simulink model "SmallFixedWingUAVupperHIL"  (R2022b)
settings: Solver=FixedStepDiscrete  StartTime=0.0  StopTime=stoptime  RelTol=1e-3
model workspace: external: MAT-File (data not in the file)
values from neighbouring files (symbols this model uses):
  env = struct    [InitDatactrl.m]
  stoptime = knots(m-pp+1)    [bspline.m]    (also in generate_poly.m = 20)
  uav = struct    [InitDatactrl.m]    (also in InitDatactrldf.m)
  x = x + points(1, i) * k(i) * ft    [bezir_n.m]
undefined symbols (not defined in the file or in its folder): current_a, current_filtered_a, DiscIntNeverNeededParam, remaining, RGBLED_COLOR_ENUM, RGBLED_MODE_ENUM, voltage_filtered_v, voltage_v
libraries: simulink x9, pixhawk_slib_sensors_actuators x4, pixhawk_slib_uORB_RW x3

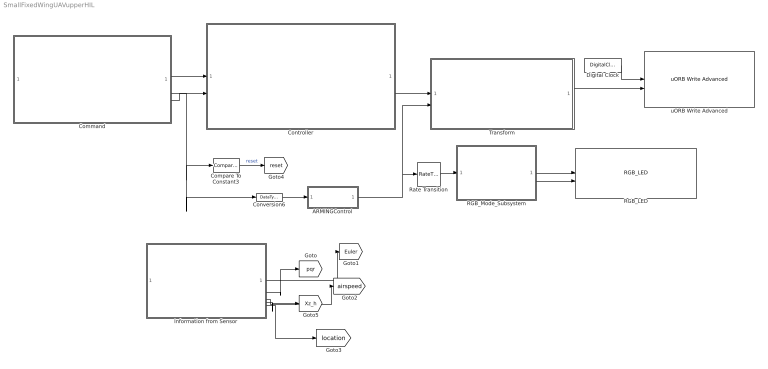
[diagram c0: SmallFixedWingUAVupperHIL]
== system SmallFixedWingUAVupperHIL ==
  ARMINGControl : Subsystem
  Command : Subsystem
  Compare To Constant3 : simulink/Logic and Bit Operations/Compare To Constant  relop=<=  const=1100  OutDataTypeStr=boolean
  Controller : Subsystem
  Conversion6 : DataTypeConversion  OutDataTypeStr=double
  Digital Clock : DigitalClock  SampleTime=-1
  Information from Sensor : Subsystem
  RGB_LED : pixhawk_slib_sensors_actuators/RGB_LED
  RGB_Mode_Subsystem : Subsystem
  Rate Transition : RateTransition  OutPortSampleTime=1
  Transform : Subsystem
  uORB Write Advanced : pixhawk_slib_uORB_RW/uORB Write Advanced  Ts=0  uORB_AdvtQueue=on  uORB_FieldEnabledArr="0  0  0  1  0  0  0  0  0  0  0"  uORB_Topic_str=0  uORB_Struct_DT="[1  1  1  1  1]"  BlockInputCount=5  uORB_StructParams="[\"voltage_v\",\"voltage_filtered_v\",\"current_a\",\"current_filtered_a\",\"remaining\"]"  uORB_PortSizes="[1  1  1  1]"  MsgSizeOf=0  MW_update=true
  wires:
  Digital Clock/1 -> uORB Write Advanced/1
  RGB_Mode_Subsystem/1(RGB_MODE) -> RGB_LED/1
  Rate Transition/1 -> RGB_Mode_Subsystem/1(ARM_STATE)
  ARMINGControl/1(Out1) -> Transform/2(In2), Rate Transition/1
  RGB_Mode_Subsystem/2(RGB_COLOR) -> RGB_LED/2
  Conversion6/1 -> ARMINGControl/1(In1)
  Compare To Constant3/1 -> [reset]  "reset"
  Transform/1(Out1) -> uORB Write Advanced/2
  Controller/1(Out1) -> Transform/1(In1)
  Command/2(Arm) -> Conversion6/1, Compare To Constant3/1
  Command/1(Command) -> Controller/1(Cmd)
  Information from Sensor/2(pqr) -> [pqr]
  Information from Sensor/4(Xz_h) -> [Xz_h]
  Information from Sensor/3(<true_airspeed_m_s>) -> [airspeed]
  Information from Sensor/1(Euler) -> [Euler]
  Information from Sensor/5(location) -> [location]
  Command/3(Command1) -> Controller/2(Cmd1)

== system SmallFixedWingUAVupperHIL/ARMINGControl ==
  In1 : Inport
  Compare To Constant3 : simulink/Logic and Bit Operations/Compare To Constant  relop=>=  const=uint16(1500)  OutDataTypeStr=boolean
  Out1 : Outport  VectorParamsAs1DForOutWhenUnconnected=off
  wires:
  Compare To Constant3/1 -> Out1/1
  In1/1 -> Compare To Constant3/1

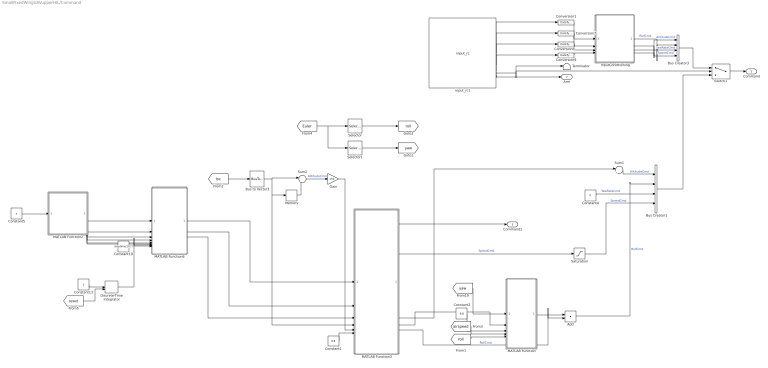
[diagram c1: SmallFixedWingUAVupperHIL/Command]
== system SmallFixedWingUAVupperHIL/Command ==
  Add : Sum
  Bus Creator1 : BusCreator  Inputs=4
  Bus Creator3 : BusCreator  Inputs=4
  Bus to Vector3 : BusToVector
  Constant1 : Constant  Value=9.8
  Constant13 : Constant  SampleTime=-1
  Constant19 : Constant  Value=stoptime/1000
  Constant2 : Constant  Value=9.8  SampleTime=-1
  Constant4 : Constant  Value=0  SampleTime=-1
  Constant5 : Constant  Value=x
  Conversion{1,7..9} (4 alike) : DataTypeConversion  OutDataTypeStr=double
  Discrete-Time Integrator : DiscreteIntegrator  ExternalReset=either  SampleTime=-1  ICPrevOutput=DiscIntNeverNeededParam  ICPrevScaledInput=DiscIntNeverNeededParam
  Gain : Gain  Gain=150
  InputConditioning : Subsystem
  MATLAB Function : MATLAB Function  TreatAsAtomicUnit=on
  MATLAB Function2 : MATLAB Function  TreatAsAtomicUnit=on
  MATLAB Function3 : MATLAB Function  TreatAsAtomicUnit=on
  MATLAB Function6 : MATLAB Function  TreatAsAtomicUnit=on
  Memory : Memory  InheritSampleTime=on
  Saturation : Saturate  UpperLimit=15  LowerLimit=10
  Selector : Selector  InputPortWidth=3  IndexOptions=Index vector (dialog)  Indices=[1]  OutputSizes=1
  Selector1 : Selector  InputPortWidth=3  IndexOptions=Index vector (dialog)  Indices=[3]  OutputSizes=1
  Sum1 : Sum  Inputs=|++
  Sum2 : Sum  Inputs=|+-
  Switch1 : Switch  Criteria=u2 > Threshold  Threshold=1500
  Terminator : Terminator
  input_rc1 : pixhawk_slib_sensors_actuators/input_rc  Description=|  sampletime=1/250  channel1=on  channel2=on  channel3=on  channel4=on  channel5=on  channel6=on  channel7=off  channel8=off  channel9=off  channel10=off  channel11=off  channel12=off  channel13=off  channel14=off  channel15=off  channel16=off  channel17=off  channel18=off  ch_count=off  rssi=off  rc_failsafe=off  rc_lost=off  rc_inputsource=off
      | RC Input Block
      | 
      | This block provides user input control to the model.
      | It uses the input_rc uORB topic.
      | 
      | The user has the ability to choose which channels are available as outputs from this block and also some optional outputs. These include 
      | Channels 1 through 18
      | double data type indicating the PWM value from the controller 
      | measured pulse widths for each of the supported channels 
      | Channel Count 
      | u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
  Command : Outport  VectorParamsAs1DForOutWhenUnconnected=off
  Arm : Outport  Port=2  VectorParamsAs1DForOutWhenUnconnected=off
  Command1 : Outport  Port=3  VectorParamsAs1DForOutWhenUnconnected=off
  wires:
  InputConditioning/3(yawRate_d) -> Bus Creator3/3  "YawRateCmd"
  input_rc1/3 -> Conversion8/1
  input_rc1/2 -> Conversion7/1
  Conversion9/1 -> InputConditioning/4(ch4)
  InputConditioning/1(Roll_d) -> Bus Creator3/2  "RollCmd"
  input_rc1/4 -> Conversion9/1
  InputConditioning/4(Speed_d) -> Bus Creator3/4  "SpeedCmd"
  Conversion1/1 -> InputConditioning/1("ch1 ")
  InputConditioning/2(Altitude_d) -> Bus Creator3/1  "AlititudeCmd"
  Conversion8/1 -> InputConditioning/3(ch3)
  input_rc1/1 -> Conversion1/1
  Conversion7/1 -> InputConditioning/2(ch2)
  Switch1/1 -> Command/1
  input_rc1/6 -> Arm/1
  MATLAB Function2/5(ddx) -> MATLAB Function6/5(ddx)
  MATLAB Function2/6(ddy) -> MATLAB Function6/6(ddy)
  Sum2/1 -> Gain/1  "AlititudeCmd"
  MATLAB Function2/2(y) -> MATLAB Function6/2(y)
  MATLAB Function6/2(vdv) -> MATLAB Function3/2(dxd)
  MATLAB Function6/1(xdx) -> MATLAB Function3/1(xd)
  MATLAB Function2/4(dy) -> MATLAB Function6/4(dy)
  [roll] -> MATLAB Function/5(rolldes)
  Constant19/1 -> MATLAB Function6/8(sample_tt)
  MATLAB Function2/1(xx) -> MATLAB Function6/1(x)
  Constant2/1 -> MATLAB Function/3(g)
  MATLAB Function2/3(dx) -> MATLAB Function6/3(dx)
  Constant5/1 -> MATLAB Function2/1(x)
  [yaw] -> MATLAB Function/1(yaw)
  Constant4/1 -> Bus Creator1/3  "YawRateCmd"
  Sum1/1 -> Bus Creator1/1  "AlititudeCmd"
  Gain/1 -> MATLAB Function3/5(dx)
  MATLAB Function3/4(yaw) -> MATLAB Function/2(yawdes)
  Saturation/1 -> Bus Creator1/4  "SpeedCmd"
  Memory/1 -> Sum2/2
  MATLAB Function6/3(ada) -> MATLAB Function3/3(ddxd)
  [airspeed] -> MATLAB Function/4(V)
  [loc] -> Bus to Vector3/1
  Bus to Vector3/1 -> Sum2/1, Memory/1, MATLAB Function3/4(x)
  input_rc1/5 -> Switch1/2, Terminator/1
  MATLAB Function/1(roll) -> Add/1
  Constant1/1 -> MATLAB Function3/6(g)
  Discrete-Time Integrator/1 -> MATLAB Function6/7(t)
  [Euler] -> Selector1/1, Selector/1
  Selector/1 -> [roll]
  Selector1/1 -> [yaw]
  Bus Creator3/1 -> Switch1/1
  [reset] -> Discrete-Time Integrator/2
  Constant13/1 -> Discrete-Time Integrator/1
  Bus Creator1/1 -> Switch1/3
  MATLAB Function3/2(va) -> Saturation/1  "SpeedCmd"
  MATLAB Function3/3(Hz) -> Sum1/1
  MATLAB Function3/1(av1) -> Command1/1
  MATLAB Function3/5(roll) -> Add/2  "RollCmd"
  Add/1 -> Bus Creator1/2  "RollCmd"

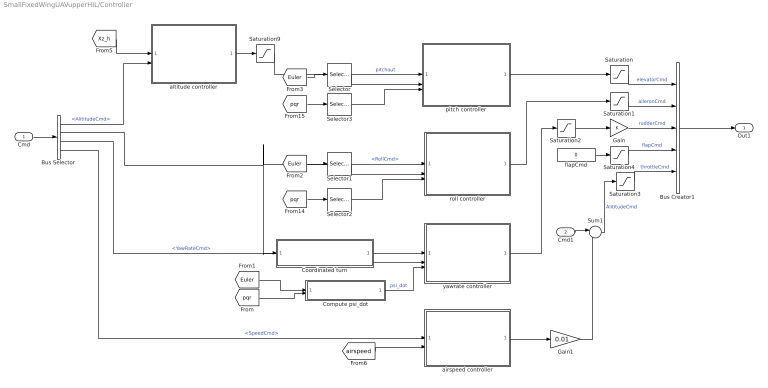
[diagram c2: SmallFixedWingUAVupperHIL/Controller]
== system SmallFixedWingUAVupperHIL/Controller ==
  Cmd : Inport
  Cmd1 : Inport  Port=2
  Bus Creator1 : BusCreator  Inputs=5
  Bus Selector : BusSelector  OutputSignals=AlititudeCmd,RollCmd,YawRateCmd,SpeedCmd
  Compute psi_dot : Subsystem
  Coordinated turn : Subsystem
  Gain : Gain
  Gain1 : Gain  Gain=0.01
  Saturation : Saturate  UpperLimit=uav.elevator.max  LowerLimit=uav.elevator.min
  Saturation1 : Saturate  UpperLimit=uav.aileron.max  LowerLimit=uav.aileron.min
  Saturation2 : Saturate  UpperLimit=uav.rudder.max  LowerLimit=uav.rudder.min
  Saturation3 : Saturate  UpperLimit=uav.throttlepercent.max  LowerLimit=uav.throttlepercent.min
  Saturation4 : Saturate  UpperLimit=uav.flap.max  LowerLimit=uav.flap.min
  Saturation9 : Saturate  UpperLimit=uav.attitudectrlmax.pitch  LowerLimit=-uav.attitudectrlmax.pitch
  Selector : Selector  InputPortWidth=3  IndexOptions=Index vector (dialog)  Indices=2  OutputSizes=1
  Selector1 : Selector  InputPortWidth=3  IndexOptions=Index vector (dialog)  Indices=1  OutputSizes=1
  Selector2 : Selector  InputPortWidth=3  IndexOptions=Index vector (dialog)  Indices=1  OutputSizes=1
  Selector3 : Selector  InputPortWidth=3  IndexOptions=Index vector (dialog)  Indices=2  OutputSizes=1
  Sum1 : Sum  Inputs=|++
  airspeed controller : Subsystem
  altitude controller : Subsystem
  flapCmd : Constant  Value=0  OutDataTypeStr=double
  pitch controller : Subsystem
  roll controller : Subsystem
  yawrate controller : Subsystem
  Out1 : Outport  VectorParamsAs1DForOutWhenUnconnected=off
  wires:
  [Euler] -> Selector/1
  Saturation9/1 -> pitch controller/1(pitchout)  "pitchout"
  Selector1/1 -> roll controller/2(phi)
  Bus Selector/4 -> airspeed controller/1(<SpeedCmd>)  "<SpeedCmd>"
  Bus Selector/3 -> yawrate controller/1(<YawRateCmd>)  "<YawRateCmd>"
  Bus Selector/1 -> altitude controller/2(<AlititudeCmd>)  "<AlititudeCmd>"
  Saturation2/1 -> Gain/1
  [pqr] -> Selector2/1
  roll controller/1(aileronCmd) -> Saturation1/1
  yawrate controller/1(rudderCmd) -> Saturation2/1
  Compute psi_dot/1(psi_dot) -> yawrate controller/3(psi_dot)  "psi_dot"
  Saturation3/1 -> Bus Creator1/5  "throttleCmd"
  Coordinated turn/1(YawRateCmd from Roll) -> yawrate controller/2(In2)
  Selector/1 -> pitch controller/2(theta)
  [Euler] -> Compute psi_dot/1(Euler)
  [airspeed] -> airspeed controller/2(airspeed)
  [Euler] -> Selector1/1
  Bus Selector/2 -> Coordinated turn/1(<RollCmd>), roll controller/1(<RollCmd>)  "<RollCmd>"
  [Xz_h] -> altitude controller/1(In1)
  Selector2/1 -> roll controller/3(p)
  Gain/1 -> Bus Creator1/3  "rudderCmd"
  [pqr] -> Selector3/1
  altitude controller/1(pitchout) -> Saturation9/1
  flapCmd/1 -> Saturation4/1
  [pqr] -> Compute psi_dot/2(G)
  Selector3/1 -> pitch controller/3(q)
  Cmd/1 -> Bus Selector/1
  Saturation/1 -> Bus Creator1/1  "elevatorCmd"
  pitch controller/1(elevatorCmd) -> Saturation/1
  Saturation4/1 -> Bus Creator1/4  "flapCmd"
  Saturation1/1 -> Bus Creator1/2  "aileronCmd"
  Bus Creator1/1 -> Out1/1
  Cmd1/1 -> Sum1/1
  Sum1/1 -> Saturation3/1  "AlititudeCmd"
  airspeed controller/1(throttleCmd) -> Gain1/1
  Gain1/1 -> Sum1/2

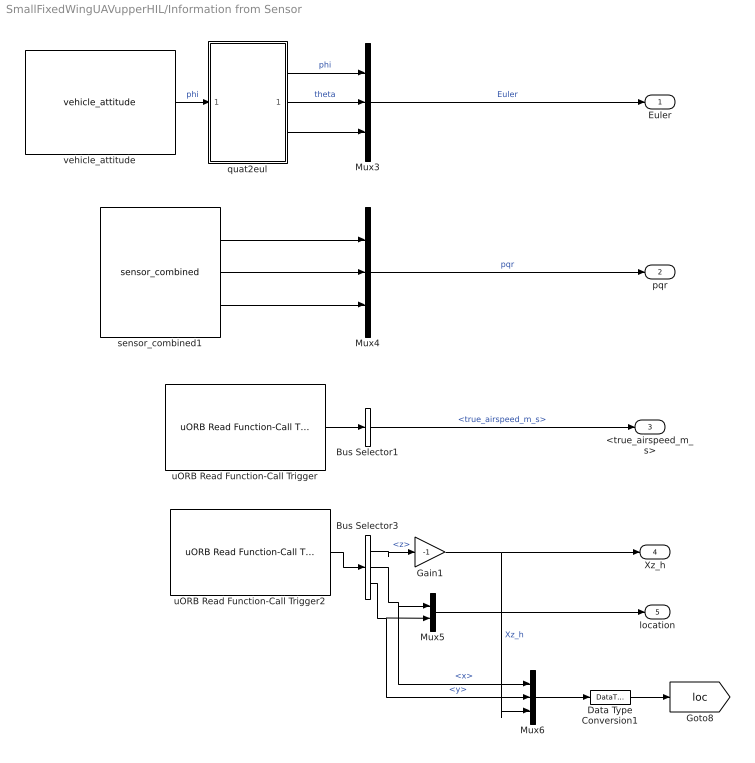
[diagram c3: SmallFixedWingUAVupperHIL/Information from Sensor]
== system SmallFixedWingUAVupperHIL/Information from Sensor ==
  Bus Selector1 : BusSelector  OutputSignals=true_airspeed_m_s
  Bus Selector3 : BusSelector  OutputSignals=z,x,y
  Data Type Conversion1 : DataTypeConversion  OutDataTypeStr=double
  Gain1 : Gain  Gain=-1
  Mux3 : Mux  Inputs=3
  Mux4 : Mux  Inputs=3
  Mux5 : Mux  Inputs=2
  Mux6 : Mux  Inputs=3
  quat2eul : MATLAB Function  TreatAsAtomicUnit=on
  sensor_combined1 : pixhawk_slib_sensors_actuators/sensor_combined  Description=|  sampletime=1/250  show_mag=off  show_acc=off  show_gyro=on  show_baro=off  show_ts=off
      | Sensor Combined Block
      | 
      | This block enables access to the various sensors available on the px4fmu-v2 hardware.  
      | The user can use these signals in the Simulink control model.  
      | The sample time needs to be provided in the mask dialog.  
      | Optional output ports can also be selected.  
      | Refer to the sample model: px4demo_attitude_control.slx
      | 
      | Signal definitions: 
      | Magnetometer (x,y,z) - single values – Mag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
  uORB Read Function-Call Trigger : pixhawk_slib_uORB_RW/uORB Read Function-Call Trigger  uORB_Topic_str='airspeed'  BusObjVar=Bus: airspeed_SL  uORB_Interval=1  AsyncOutput=off  Fcn_call_select=Generate Function Call Signal  TaskName='Task1'  Poll_timeout=100  Ts=-1
  uORB Read Function-Call Trigger2 : pixhawk_slib_uORB_RW/uORB Read Function-Call Trigger  uORB_Topic_str='vehicle_local_position'  BusObjVar=Bus: vehicle_local_position_SL  uORB_Interval=1  AsyncOutput=off  Fcn_call_select=Generate Function Call Signal  TaskName='Task1'  Poll_timeout=100  Ts=-1
  vehicle_attitude : pixhawk_slib_sensors_actuators/vehicle_attitude  sampletime=1/250  show_r=off  show_p=off  show_y=off  show_q=on  show_ts=off
  Euler : Outport  VectorParamsAs1DForOutWhenUnconnected=off
  pqr : Outport  Port=2  VectorParamsAs1DForOutWhenUnconnected=off
  <true_airspeed_m_s> : Outport  Port=3  VectorParamsAs1DForOutWhenUnconnected=off
  Xz_h : Outport  Port=4  VectorParamsAs1DForOutWhenUnconnected=off
  location : Outport  Port=5  VectorParamsAs1DForOutWhenUnconnected=off
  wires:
  vehicle_attitude/1 -> quat2eul/1(q)  "phi"
  quat2eul/2(theta) -> Mux3/2  "theta"
  quat2eul/3(psi) -> Mux3/3
  sensor_combined1/3 -> Mux4/3
  Bus Selector3/1 -> Gain1/1  "<z>"
  sensor_combined1/1 -> Mux4/1
  uORB Read Function-Call Trigger/1 -> Bus Selector1/1
  uORB Read Function-Call Trigger2/1 -> Bus Selector3/1
  Mux4/1 -> pqr/1  "pqr"
  quat2eul/1(phi) -> Mux3/1  "phi"
  Bus Selector1/1 -> <true_airspeed_m_s>/1  "<true_airspeed_m_s>"
  sensor_combined1/2 -> Mux4/2
  Mux3/1 -> Euler/1  "Euler"
  Mux5/1 -> location/1
  Bus Selector3/3 -> Mux6/2, Mux5/2  "<y>"
  Data Type Conversion1/1 -> [loc]
  Mux6/1 -> Data Type Conversion1/1
  Gain1/1 -> Xz_h/1, Mux6/3  "Xz_h"
  Bus Selector3/2 -> Mux6/1, Mux5/1  "<x>"

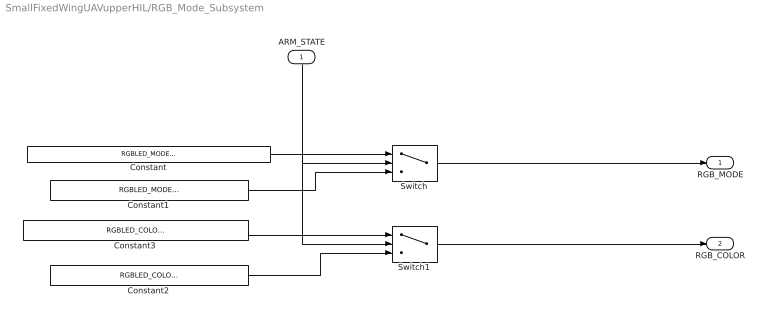
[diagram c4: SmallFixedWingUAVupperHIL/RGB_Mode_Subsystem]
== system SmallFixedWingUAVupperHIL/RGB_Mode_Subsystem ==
  ARM_STATE : Inport
  Constant : Constant  Value=RGBLED_MODE_ENUM.SL_MODE_BLINK_FAST  OutDataTypeStr=Enum: RGBLED_MODE_ENUM
  Constant1 : Constant  Value=RGBLED_MODE_ENUM.SL_MODE_BREATHE  OutDataTypeStr=Enum: RGBLED_MODE_ENUM
  Constant2 : Constant  Value=RGBLED_COLOR_ENUM.SL_COLOR_GREEN  OutDataTypeStr=Enum: RGBLED_COLOR_ENUM
  Constant3 : Constant  Value=RGBLED_COLOR_ENUM.SL_COLOR_BLUE  OutDataTypeStr=Enum: RGBLED_COLOR_ENUM
  Switch : Switch  Criteria=u2 ~= 0  Threshold=1500
  Switch1 : Switch  Criteria=u2 ~= 0  Threshold=1500
  RGB_MODE : Outport  VectorParamsAs1DForOutWhenUnconnected=off
  RGB_COLOR : Outport  Port=2  VectorParamsAs1DForOutWhenUnconnected=off
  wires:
  ARM_STATE/1 -> Switch1/2, Switch/2
  Constant/1 -> Switch/1
  Constant1/1 -> Switch/3
  Switch/1 -> RGB_MODE/1
  Constant3/1 -> Switch1/1
  Constant2/1 -> Switch1/3
  Switch1/1 -> RGB_COLOR/1

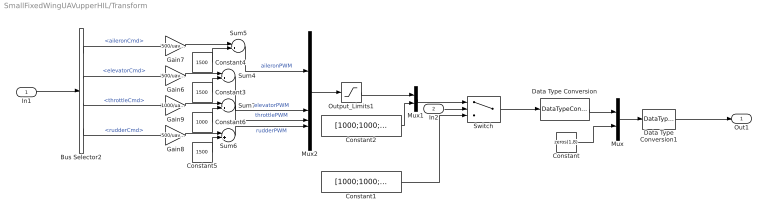
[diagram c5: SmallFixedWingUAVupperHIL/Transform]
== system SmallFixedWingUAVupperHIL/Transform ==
  In1 : Inport
  In2 : Inport  Port=2
  Bus Selector2 : BusSelector  OutputSignals=aileronCmd,elevatorCmd,throttleCmd,rudderCmd
  Constant : Constant  Value=zeros(1,8)
  Constant1 : Constant  Value=[1000;1000;1000;1000;1000;1000;1000;1000]
  Constant2 : Constant  Value=[1000;1000;1000;1000]
  Constant3 : Constant  Value=1500
  Constant4 : Constant  Value=1500
  Constant5 : Constant  Value=1500
  Constant6 : Constant  Value=1000
  Data Type Conversion : DataTypeConversion  OutDataTypeStr=double
  Data Type Conversion1 : DataTypeConversion  OutDataTypeStr=single
  Gain6 : Gain  Gain=500/uav.controlsurfacemax
  Gain7 : Gain  Gain=500/uav.controlsurfacemax
  Gain8 : Gain  Gain=500/uav.controlsurfacemax
  Gain9 : Gain  Gain=1000/uav.throttlepercent.max
  Mux : Mux  Inputs=2
  Mux1 : Mux  Inputs=2
  Mux2 : Mux
  Output_Limits1 : Saturate  UpperLimit=2000  LowerLimit=1000
  Sum{4..7} (4 alike) : Sum  Inputs=|++
  Switch : Switch  Criteria=u2 > Threshold  Threshold=0.5
  Out1 : Outport  VectorParamsAs1DForOutWhenUnconnected=off
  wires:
  Constant2/1 -> Mux1/2
  Sum6/1 -> Mux2/4  "rudderPWM"
  Data Type Conversion/1 -> Mux/1
  Bus Selector2/4 -> Gain8/1  "<rudderCmd>"
  Bus Selector2/2 -> Gain6/1  "<elevatorCmd>"
  Constant3/1 -> Sum4/2
  Switch/1 -> Data Type Conversion/1
  Gain6/1 -> Sum4/1
  Bus Selector2/3 -> Gain9/1  "<throttleCmd>"
  Bus Selector2/1 -> Gain7/1  "<aileronCmd>"
  Constant/1 -> Mux/2
  Gain8/1 -> Sum6/1
  Sum7/1 -> Mux2/3  "throttlePWM"
  Constant1/1 -> Switch/3
  Mux1/1 -> Switch/1
  Output_Limits1/1 -> Mux1/1
  Constant5/1 -> Sum6/2
  Sum5/1 -> Mux2/1  "aileronPWM"
  Sum4/1 -> Mux2/2  "elevatorPWM"
  Constant6/1 -> Sum7/2
  Mux2/1 -> Output_Limits1/1
  Gain7/1 -> Sum5/1
  Mux/1 -> Data Type Conversion1/1
  Gain9/1 -> Sum7/1
  Constant4/1 -> Sum5/2
  In2/1 -> Switch/2
  In1/1 -> Bus Selector2/1
  Data Type Conversion1/1 -> Out1/1

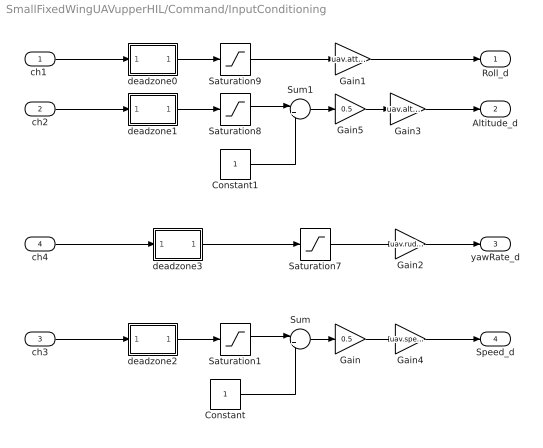
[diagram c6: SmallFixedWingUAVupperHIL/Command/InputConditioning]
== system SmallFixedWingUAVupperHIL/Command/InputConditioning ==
  "ch1 " : Inport
  ch2 : Inport  Port=2
  ch3 : Inport  Port=3
  ch4 : Inport  Port=4
  Constant : Constant
  Constant1 : Constant
  Gain : Gain  Gain=0.5
  Gain1 : Gain  Gain=uav.attitudectrlmax.roll  OutDataTypeStr=Inherit: Inherit via back propagation
  Gain2 : Gain  Gain=uav.rudder.max
  Gain3 : Gain  Gain=uav.altitude.max  OutDataTypeStr=Inherit: Inherit via back propagation
  Gain4 : Gain  Gain=uav.speed.max
  Gain5 : Gain  Gain=0.5
  Saturation{1,7..9} (4 alike) : Saturate  UpperLimit=1  LowerLimit=-1
  Sum : Sum  Inputs=|++
  Sum1 : Sum  Inputs=|++
  deadzone0 : MATLAB Function  TreatAsAtomicUnit=on
  deadzone1 : MATLAB Function  TreatAsAtomicUnit=on
  deadzone2 : MATLAB Function  TreatAsAtomicUnit=on
  deadzone3 : MATLAB Function  TreatAsAtomicUnit=on
  Roll_d : Outport  VectorParamsAs1DForOutWhenUnconnected=off
  Altitude_d : Outport  Port=2  VectorParamsAs1DForOutWhenUnconnected=off
  yawRate_d : Outport  Port=3  VectorParamsAs1DForOutWhenUnconnected=off
  Speed_d : Outport  Port=4  VectorParamsAs1DForOutWhenUnconnected=off
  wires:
  deadzone2/1(y) -> Saturation1/1
  ch3/1 -> deadzone2/1(u)
  deadzone1/1(y) -> Saturation8/1
  Gain/1 -> Gain4/1
  deadzone0/1(y) -> Saturation9/1
  "ch1 "/1 -> deadzone0/1(u)
  ch2/1 -> deadzone1/1(u)
  Saturation9/1 -> Gain1/1
  Saturation8/1 -> Sum1/1
  Constant/1 -> Sum/2
  Sum/1 -> Gain/1
  Gain1/1 -> Roll_d/1
  Gain3/1 -> Altitude_d/1
  Saturation7/1 -> Gain2/1
  deadzone3/1(y) -> Saturation7/1
  ch4/1 -> deadzone3/1(u)
  Gain2/1 -> yawRate_d/1
  Saturation1/1 -> Sum/1
  Gain4/1 -> Speed_d/1
  Gain5/1 -> Gain3/1
  Constant1/1 -> Sum1/2
  Sum1/1 -> Gain5/1

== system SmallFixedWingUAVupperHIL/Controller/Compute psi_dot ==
  Euler : Inport
  G : Inport  Port=2
  Mux1 : Mux  Inputs=2
  psidot : Fcn  Expr=(u[5]*sin(u[1])+u[6]*cos(u[1]))/cos(u[2])
  psi_dot : Outport  Unit=rad/S  VectorParamsAs1DForOutWhenUnconnected=off
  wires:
  G/1 -> Mux1/2
  psidot/1 -> psi_dot/1  "psi_dot"
  Mux1/1 -> psidot/1
  Euler/1 -> Mux1/1

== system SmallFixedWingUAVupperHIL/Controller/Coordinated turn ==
  <RollCmd> : Inport
  Divide : Product  Inputs=*/*
  Trigonometric Function : Trigonometry  Operator=tan
  env.ISA_g : Constant  Value=env.ISA_g
  YawRateCmd from Roll : Outport  VectorParamsAs1DForOutWhenUnconnected=off
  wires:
  env.ISA_g/1 -> Divide/3
  [airspeed] -> Divide/2
  Trigonometric Function/1 -> Divide/1
  Divide/1 -> YawRateCmd from Roll/1  "YawRateCmd from Roll"
  <RollCmd>/1 -> Trigonometric Function/1

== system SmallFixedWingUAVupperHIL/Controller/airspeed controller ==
  <SpeedCmd> : Inport
  airspeed : Inport  Port=2
  Add7 : Sum  Inputs=+-
  PID_Speed : Subsystem
  throttleCmd : Outport  VectorParamsAs1DForOutWhenUnconnected=off
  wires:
  [reset] -> PID_Speed/2(reset_i)
  airspeed/1 -> Add7/2
  Add7/1 -> PID_Speed/1(x)  "speederror"
  PID_Speed/1(y) -> throttleCmd/1
  <SpeedCmd>/1 -> Add7/1

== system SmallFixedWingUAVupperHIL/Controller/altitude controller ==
  In1 : Inport
  <AlititudeCmd> : Inport  Port=2
  Add8 : Sum  Inputs=+-
  PID_Altitude : Subsystem
  pitchout : Outport  VectorParamsAs1DForOutWhenUnconnected=off
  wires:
  [reset] -> PID_Altitude/2(reset_i)
  In1/1 -> Add8/2
  Add8/1 -> PID_Altitude/1(x)
  <AlititudeCmd>/1 -> Add8/1
  PID_Altitude/1(y) -> pitchout/1  "pitchout"

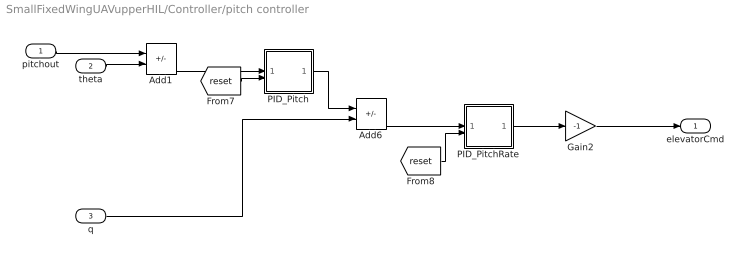
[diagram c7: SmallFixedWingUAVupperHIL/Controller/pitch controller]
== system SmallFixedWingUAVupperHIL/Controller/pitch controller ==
  pitchout : Inport
  theta : Inport  Port=2
  q : Inport  Port=3
  Add1 : Sum  Inputs=+-
  Add6 : Sum  Inputs=+-
  Gain2 : Gain  Gain=-1
  PID_Pitch : Subsystem
  PID_PitchRate : Subsystem
  elevatorCmd : Outport  VectorParamsAs1DForOutWhenUnconnected=off
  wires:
  PID_PitchRate/1(y) -> Gain2/1
  q/1 -> Add6/2
  Add1/1 -> PID_Pitch/1(x)
  [reset] -> PID_PitchRate/2(reset_i)
  [reset] -> PID_Pitch/2(reset_i)
  theta/1 -> Add1/2
  PID_Pitch/1(y) -> Add6/1
  Add6/1 -> PID_PitchRate/1(x)
  Gain2/1 -> elevatorCmd/1
  pitchout/1 -> Add1/1

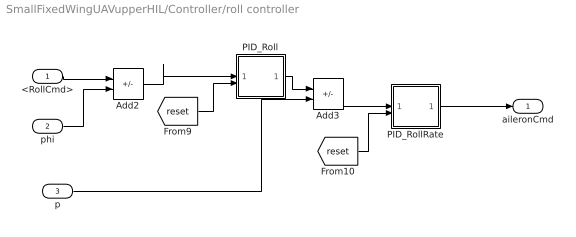
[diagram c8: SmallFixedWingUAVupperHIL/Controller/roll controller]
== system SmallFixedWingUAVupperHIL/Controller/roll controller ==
  <RollCmd> : Inport
  phi : Inport  Port=2
  p : Inport  Port=3
  Add2 : Sum  Inputs=+-
  Add3 : Sum  Inputs=+-
  PID_Roll : Subsystem
  PID_RollRate : Subsystem
  aileronCmd : Outport  VectorParamsAs1DForOutWhenUnconnected=off
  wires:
  Add3/1 -> PID_RollRate/1(x)
  [reset] -> PID_Roll/2(reset_i)
  PID_Roll/1(y) -> Add3/1
  Add2/1 -> PID_Roll/1(x)
  [reset] -> PID_RollRate/2(reset_i)
  PID_RollRate/1(y) -> aileronCmd/1
  phi/1 -> Add2/2
  p/1 -> Add3/2
  <RollCmd>/1 -> Add2/1

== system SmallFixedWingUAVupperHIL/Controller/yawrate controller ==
  <YawRateCmd> : Inport
  In2 : Inport  Port=2
  psi_dot : Inport  Port=3
  Add4 : Sum  Inputs=+-
  PID_YawRate : Subsystem
  Sum2 : Sum  Inputs=++|
  rudderCmd : Outport  VectorParamsAs1DForOutWhenUnconnected=off
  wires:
  Add4/1 -> PID_YawRate/1(x)
  [reset] -> PID_YawRate/2(reset_i)
  psi_dot/1 -> Add4/2
  PID_YawRate/1(y) -> Sum2/2
  <YawRateCmd>/1 -> Sum2/1
  Sum2/1 -> rudderCmd/1
  In2/1 -> Add4/1

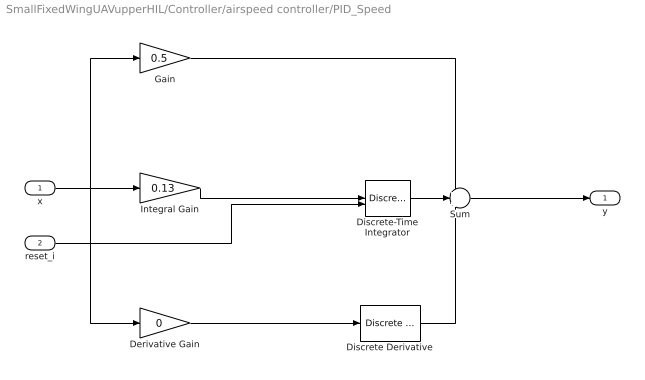
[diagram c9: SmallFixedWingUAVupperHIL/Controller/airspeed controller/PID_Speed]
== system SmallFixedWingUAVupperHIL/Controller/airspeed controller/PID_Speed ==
  x : Inport
  reset_i : Inport  Port=2
  Derivative Gain : Gain  DisableCoverage=on  Gain=0  ParamMin=-100  ParamMax=100  OutMin=-100  OutMax=100
  Discrete Derivative : simulink/Discrete/Discrete Derivative  gainval=1.0  ICPrevScaledInput=0.0  OutMin=[]  OutMax=[]  OutDataType=fixdt(1, 16)  OutScaling=2^-10  DoSatur=off
  Discrete-Time Integrator : DiscreteIntegrator  ExternalReset=either  SampleTime=-1  UpperSaturationLimit=0.3  LowerSaturationLimit=-0.3  ICPrevOutput=DiscIntNeverNeededParam  ICPrevScaledInput=DiscIntNeverNeededParam
  Gain : Gain  Gain=0.5
  Integral Gain : Gain  DisableCoverage=on  Gain=0.13
  Sum : Sum  Inputs=+++
  y : Outport  InitialOutput=0  VectorParamsAs1DForOutWhenUnconnected=off
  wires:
  reset_i/1 -> Discrete-Time Integrator/2
  Discrete-Time Integrator/1 -> Sum/2
  Discrete Derivative/1 -> Sum/3
  Sum/1 -> y/1
  Gain/1 -> Sum/1
  Derivative Gain/1 -> Discrete Derivative/1
  Integral Gain/1 -> Discrete-Time Integrator/1
  x/1 -> Derivative Gain/1, Integral Gain/1, Gain/1

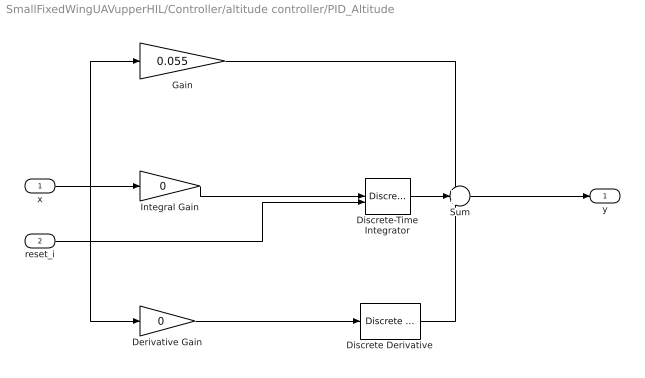
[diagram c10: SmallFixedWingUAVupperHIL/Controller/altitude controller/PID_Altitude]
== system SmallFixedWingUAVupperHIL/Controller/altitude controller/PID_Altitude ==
  x : Inport
  reset_i : Inport  Port=2
  Derivative Gain : Gain  DisableCoverage=on  Gain=0  ParamMin=-100  ParamMax=100  OutMin=-100  OutMax=100
  Discrete Derivative : simulink/Discrete/Discrete Derivative  gainval=1.0  ICPrevScaledInput=0.0  OutMin=[]  OutMax=[]  OutDataType=fixdt(1, 16)  OutScaling=2^-10  DoSatur=off
  Discrete-Time Integrator : DiscreteIntegrator  ExternalReset=either  SampleTime=-1  ICPrevOutput=DiscIntNeverNeededParam  ICPrevScaledInput=DiscIntNeverNeededParam
  Gain : Gain  Gain=0.055
  Integral Gain : Gain  DisableCoverage=on  Gain=0
  Sum : Sum  Inputs=+++
  y : Outport  InitialOutput=0  VectorParamsAs1DForOutWhenUnconnected=off
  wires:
  x/1 -> Gain/1, Integral Gain/1, Derivative Gain/1
  Integral Gain/1 -> Discrete-Time Integrator/1
  Derivative Gain/1 -> Discrete Derivative/1
  Gain/1 -> Sum/1
  Sum/1 -> y/1
  Discrete Derivative/1 -> Sum/3
  Discrete-Time Integrator/1 -> Sum/2
  reset_i/1 -> Discrete-Time Integrator/2

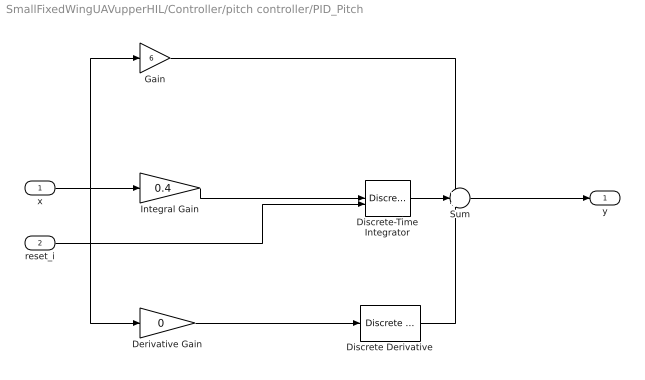
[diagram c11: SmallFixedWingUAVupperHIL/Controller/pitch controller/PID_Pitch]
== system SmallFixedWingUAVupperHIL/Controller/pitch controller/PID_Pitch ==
  x : Inport
  reset_i : Inport  Port=2
  Derivative Gain : Gain  DisableCoverage=on  Gain=0  ParamMin=-100  ParamMax=100  OutMin=-100  OutMax=100
  Discrete Derivative : simulink/Discrete/Discrete Derivative  gainval=1.0  ICPrevScaledInput=0.0  OutMin=[]  OutMax=[]  OutDataType=fixdt(1, 16)  OutScaling=2^-10  DoSatur=off
  Discrete-Time Integrator : DiscreteIntegrator  ExternalReset=either  SampleTime=-1  ICPrevOutput=DiscIntNeverNeededParam  ICPrevScaledInput=DiscIntNeverNeededParam
  Gain : Gain  Gain=6
  Integral Gain : Gain  DisableCoverage=on  Gain=0.4
  Sum : Sum  Inputs=+++
  y : Outport  InitialOutput=0  VectorParamsAs1DForOutWhenUnconnected=off
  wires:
  reset_i/1 -> Discrete-Time Integrator/2
  Discrete-Time Integrator/1 -> Sum/2
  Discrete Derivative/1 -> Sum/3
  Sum/1 -> y/1
  Gain/1 -> Sum/1
  Derivative Gain/1 -> Discrete Derivative/1
  Integral Gain/1 -> Discrete-Time Integrator/1
  x/1 -> Derivative Gain/1, Integral Gain/1, Gain/1

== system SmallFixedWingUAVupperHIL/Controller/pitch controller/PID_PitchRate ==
  x : Inport
  reset_i : Inport  Port=2
  Derivative Gain : Gain  DisableCoverage=on  Gain=0.04  ParamMin=-100  ParamMax=100  OutMin=-100  OutMax=100
  Discrete Derivative : simulink/Discrete/Discrete Derivative  gainval=1.0  ICPrevScaledInput=0.0  OutMin=[]  OutMax=[]  OutDataType=fixdt(1, 16)  OutScaling=2^-10  DoSatur=off
  Discrete-Time Integrator : DiscreteIntegrator  ExternalReset=either  SampleTime=-1  LimitOutput=on  UpperSaturationLimit=0.3  LowerSaturationLimit=-0.3  ICPrevOutput=DiscIntNeverNeededParam  ICPrevScaledInput=DiscIntNeverNeededParam
  Gain : Gain  Gain=0.8
  Integral Gain : Gain  DisableCoverage=on  Gain=12
  Sum : Sum  Inputs=+++
  y : Outport  InitialOutput=0  VectorParamsAs1DForOutWhenUnconnected=off
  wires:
  x/1 -> Gain/1, Integral Gain/1, Derivative Gain/1
  Integral Gain/1 -> Discrete-Time Integrator/1
  Derivative Gain/1 -> Discrete Derivative/1
  Gain/1 -> Sum/1
  Sum/1 -> y/1
  Discrete Derivative/1 -> Sum/3
  Discrete-Time Integrator/1 -> Sum/2
  reset_i/1 -> Discrete-Time Integrator/2

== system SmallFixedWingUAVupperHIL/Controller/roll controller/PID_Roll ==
  x : Inport
  reset_i : Inport  Port=2
  Derivative Gain : Gain  DisableCoverage=on  Gain=0  ParamMin=-100  ParamMax=100  OutMin=-100  OutMax=100
  Discrete Derivative : simulink/Discrete/Discrete Derivative  gainval=1.0  ICPrevScaledInput=0.0  OutMin=[]  OutMax=[]  OutDataType=fixdt(1, 16)  OutScaling=2^-10  DoSatur=off
  Discrete-Time Integrator : DiscreteIntegrator  ExternalReset=either  SampleTime=-1  ICPrevOutput=DiscIntNeverNeededParam  ICPrevScaledInput=DiscIntNeverNeededParam
  Gain : Gain  Gain=9
  Integral Gain : Gain  DisableCoverage=on  Gain=0.4
  Sum : Sum  Inputs=+++
  y : Outport  InitialOutput=0  VectorParamsAs1DForOutWhenUnconnected=off
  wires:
  x/1 -> Gain/1, Integral Gain/1, Derivative Gain/1
  Integral Gain/1 -> Discrete-Time Integrator/1
  Derivative Gain/1 -> Discrete Derivative/1
  Gain/1 -> Sum/1
  Sum/1 -> y/1
  Discrete Derivative/1 -> Sum/3
  Discrete-Time Integrator/1 -> Sum/2
  reset_i/1 -> Discrete-Time Integrator/2

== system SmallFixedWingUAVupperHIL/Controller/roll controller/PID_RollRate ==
  x : Inport
  reset_i : Inport  Port=2
  Derivative Gain : Gain  DisableCoverage=on  Gain=0.01  ParamMin=-100  ParamMax=100  OutMin=-100  OutMax=100
  Discrete Derivative : simulink/Discrete/Discrete Derivative  gainval=1.0  ICPrevScaledInput=0.0  OutMin=[]  OutMax=[]  OutDataType=fixdt(1, 16)  OutScaling=2^-10  DoSatur=off
  Discrete-Time Integrator : DiscreteIntegrator  ExternalReset=either  SampleTime=-1  LimitOutput=on  UpperSaturationLimit=0.3  LowerSaturationLimit=-0.3  ICPrevOutput=DiscIntNeverNeededParam  ICPrevScaledInput=DiscIntNeverNeededParam
  Gain : Gain  Gain=0.8
  Integral Gain : Gain  DisableCoverage=on  Gain=2
  Sum : Sum  Inputs=+++
  y : Outport  InitialOutput=0  VectorParamsAs1DForOutWhenUnconnected=off
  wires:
  reset_i/1 -> Discrete-Time Integrator/2
  Discrete-Time Integrator/1 -> Sum/2
  Discrete Derivative/1 -> Sum/3
  Sum/1 -> y/1
  Gain/1 -> Sum/1
  Derivative Gain/1 -> Discrete Derivative/1
  Integral Gain/1 -> Discrete-Time Integrator/1
  x/1 -> Derivative Gain/1, Integral Gain/1, Gain/1

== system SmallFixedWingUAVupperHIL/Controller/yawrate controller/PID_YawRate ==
  x : Inport
  reset_i : Inport  Port=2
  Derivative Gain : Gain  DisableCoverage=on  Gain=0.3  ParamMin=-100  ParamMax=100  OutMin=-100  OutMax=100
  Discrete Derivative : simulink/Discrete/Discrete Derivative  gainval=1.0  ICPrevScaledInput=0.0  OutMin=[]  OutMax=[]  OutDataType=fixdt(1, 16)  OutScaling=2^-10  DoSatur=off
  Discrete-Time Integrator : DiscreteIntegrator  ExternalReset=either  SampleTime=-1  LimitOutput=on  UpperSaturationLimit=0.3  LowerSaturationLimit=-0.3  ICPrevOutput=DiscIntNeverNeededParam  ICPrevScaledInput=DiscIntNeverNeededParam
  Gain : Gain  Gain=4
  Integral Gain : Gain  DisableCoverage=on  Gain=3
  Sum : Sum  Inputs=+++
  y : Outport  InitialOutput=0  VectorParamsAs1DForOutWhenUnconnected=off
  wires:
  x/1 -> Gain/1, Integral Gain/1, Derivative Gain/1
  Integral Gain/1 -> Discrete-Time Integrator/1
  Derivative Gain/1 -> Discrete Derivative/1
  Gain/1 -> Sum/1
  Sum/1 -> y/1
  Discrete Derivative/1 -> Sum/3
  Discrete-Time Integrator/1 -> Sum/2
  reset_i/1 -> Discrete-Time Integrator/2

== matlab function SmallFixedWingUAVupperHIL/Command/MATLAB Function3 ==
function [av1,va,Hz,yaw,roll] = DF(xd,dxd,ddxd,x,dx,g)
    av1 = (0); 
    Hz= (0); 
    yaw= (0); 
    roll= (0); 
    va = (0);

    xd = [xd(1);xd(2);xd(3)];
    dxd = [dxd(1);dxd(2);dxd(3)];
    ddxd = [ddxd(1);ddxd(2);ddxd(3)];
    x = [x(1);x(2);x(3)];
    dx = [dx(1);dx(2);dx(3)];
%     x1 = (xd-x)/norm(xd-x);
    r1 = zeros(3,1);
    r1 = (dxd+0.2*(xd-x))/(norm(dxd+0.2*(xd-x))+0.001);
    
    va = norm(dxd);


    av1 = ( r1'*(1*ddxd-[0;0;g]+5*(dxd-dx)+3*(xd-x)));
     %%
%     t1 = zeros(3,1,'single');
%     t2 = zeros(3,1,'single');
%     t3 = zeros(3,1,'single');
%     t4 = zeros(3,1,'single');
%     t1(1,1) = ddxd(1,1);
%     t1(2,1) = ddxd(2,1);
%     t1(3,1) = ddxd(3,1) - single(g);
%     
%     for i = 1:3
%     t2(i,1) = single(3) * (dxd(i,1) - dx(i,1));
%     t3(i,1) = single(0.1) * (xd(i,1) - x(i,1));
% 
%     end
% 
%     for i = 1:3
%     t4(i,1) = t1(i,1) + t2(i,1) + t3(i,1);
%     end
%     av1 = single( r1'*t4);
%%

    an = (eye(3)-(r1*r1'))*((ddxd)-([0;0;g]));

    av3 = -(norm(an));
    
    Hz = (xd(3));


    r3 = (an)/((av3)+(0.001));

    r2 = cross(r3,r1);

    yaw = (atan2(r1(2),r1(1)));
    
    roll = 1*(atan2(r2(3),r3(3)));

    if isnan(av1)
        av1=(0);
    end
    if isnan(Hz)
        Hz=(0);
    end
    if isnan(yaw)
        yaw=(0);
    end

end

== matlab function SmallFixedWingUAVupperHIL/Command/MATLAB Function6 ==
function [xdx,vdv,ada]  = track(x,y,dx,dy,ddx,ddy,t,sample_tt)
%     xdx = [0;0;0];
%     vdv = [0;0;0];
%     ada = [0;0;0];
%     if (t>10)
%         t = t-10;
    index = int16(t/sample_tt);
    if index <= 1
        index = int16(1);
    end
    if index >= length(x)
        index = int16(length(x));
    end
    xx = x(index);
    yy = y(index);
    dxx = dx(index);
    dyy = dy(index);
    ddxx = ddx(index);
    ddyy = ddy(index);

    xdx = [xx;-yy;50];
    vdv = [dxx;-dyy;0];
    ada = [ddxx;-ddyy;0];
%     end

end

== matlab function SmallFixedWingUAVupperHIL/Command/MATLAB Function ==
function roll = fcn(yaw,yawdes,g,V,rolldes)
%     roll = yawrate*g*V;
    if yaw>pi
        yaw = yaw-2*pi;
    end
    yawrate = 0.5*(yawdes-yaw);
    roll = atan2(V.*yawrate,g);
end

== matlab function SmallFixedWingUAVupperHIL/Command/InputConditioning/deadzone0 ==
function y = fcn(u)
%Function description:
%  Control the range of the remote control input from RCMin to RCMax,which can be obtained from QGC. And set
%  a dead zone with a dead zone size of deadZone,the output y is normalized to 0~1.
RCMin = 1100;
RCMax = 1900;
RCMid = (RCMin + RCMax)/2;
deadZoneRate = 0.05;
deadZone = deadZoneRate*(RCMax - RCMin);
k = 1/(RCMax - RCMid - deadZone);
%Limiting
if(u < RCMin)
    u = RCMin;
elseif(u > RCMax)
    u = RCMax;
end
%dead zone and normalize
 if(u > RCMid + deadZone)
    y = (u-RCMid - deadZone)*k;
 elseif(u < RCMid - deadZone)
     y = (u - RCMid + deadZone)*k;
 else
     y = 0;
 end

 end

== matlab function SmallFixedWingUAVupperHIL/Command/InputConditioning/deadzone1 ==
function y = fcn(u)
%Function description:
%  Control the range of the remote control input from RCMin to RCMax, and set
%  a dead zone with a dead zone size of ±deadZone,the output y is
%  normalized to 0~1.You can get the RC calibration parameters in QGC.
RCMin = 1100;
RCMax = 1900;
RCMid = (RCMin + RCMax)/2;
deadZoneRate = 0.05;
deadZone = deadZoneRate*(RCMax - RCMin);
k = 1/(RCMax - RCMid - deadZone);
%Limiting
if(u < RCMin)
    u = RCMin;
elseif(u > RCMax)
    u = RCMax;
end
%dead zone and normalize
 if(u > RCMid + deadZone)
    y = (u-RCMid - deadZone)*k;
 elseif(u < RCMid - deadZone)
     y = (u - RCMid + deadZone)*k;
 else
     y = 0;
 end

 end

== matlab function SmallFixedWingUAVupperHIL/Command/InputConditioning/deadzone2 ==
function y = fcn(u)
%Function description:
%  Control the range of the remote control input from RCMin to RCMax, and set
%  a dead zone with a dead zone size of ±deadZone,the output y is
%  normalized to 0~1.You can get the RC calibration parameters in QGC.
RCMin = 1100;
RCMax = 1900;
RCMid = (RCMin + RCMax)/2;
deadZoneRate = 0.05;
deadZone = deadZoneRate*(RCMax - RCMin);
k = 1/(RCMax - RCMid - deadZone);
%Limiting
if(u < RCMin)
    u = RCMin;
elseif(u > RCMax)
    u = RCMax;
end
%dead zone and normalize
 if(u > RCMid + deadZone)
    y = (u-RCMid - deadZone)*k;
 elseif(u < RCMid - deadZone)
     y = (u - RCMid + deadZone)*k;
 else
     y = 0;
 end

 end

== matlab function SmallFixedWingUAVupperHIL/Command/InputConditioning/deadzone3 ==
function y = fcn(u)
%Function description:
%  Control the range of the remote control input from RCMin to RCMax, and set
%  a dead zone with a dead zone size of ±deadZone,the output y is
%  normalized to 0~1.You can get the RC calibration parameters in QGC.
RCMin = 1100;
RCMax = 1900;
RCMid = (RCMin + RCMax)/2;
deadZoneRate = 0.05;
deadZone = deadZoneRate*(RCMax - RCMin);
k = 1/(RCMax - RCMid - deadZone);
%Limiting
if(u < RCMin)
    u = RCMin;
elseif(u > RCMax)
    u = RCMax;
end
%dead zone and normalize
 if(u > RCMid + deadZone)
    y = (u-RCMid - deadZone)*k;
 elseif(u < RCMid - deadZone)
     y = (u - RCMid + deadZone)*k;
 else
     y = 0;
 end

 end

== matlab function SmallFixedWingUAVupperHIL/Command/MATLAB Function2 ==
function [xx,y,dx,dy,ddx,ddy]  = track(x)
%     index = int8(t/sample_tt);
%     if index <= 1
%         index = int8(1);
%     end
%     if index >= length(x)
%         index = int8(length(x));
%     end
    len = length(x)/6;

    xx = x(1:len);
    y = x(len+1:2*len);
    dx = x(2*len+1:3*len);
    dy = x(3*len+1:4*len);
    ddx = x(4*len+1:5*len);
    ddy = x(5*len+1:6*len);
end

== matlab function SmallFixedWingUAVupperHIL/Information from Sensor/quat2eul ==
function [phi,theta,psi] = quat2eul(q)
% Conversion from Quaternion to Euler angles based on the PX4 Firmware
% v1.6.5 release.
% 
% Quaternion -> DCM -> Euler Angles
% INPUT:
%   q: Quaternion vector of the format: (a + bi + cj + dk)
% OUTPUT:
%   [phi,theta,psi]: Euler angles in radians.
% 
 
    a = q(1);
    b = q(2);
    c = q(3);
    d = q(4);

    aSq = a*a;
    bSq = b*b;
    cSq = c*c;
    dSq = d*d;

    d_pi2 = pi/2;

    % quaternion_to_dcm
    dcm00 = aSq + bSq - cSq - dSq;
    % dcm01 = 2*(b*c - a*d);
    dcm02 = 2*(a*c + b*d);
    dcm10 = 2*(b*c + a*d);
    % dcm11 = aSq - bSq + cSq - dSq;
    dcm12 = 2*(c*d - a*b);
    dcm20 = 2*(b*d - a*c);
    dcm21 = 2*(a*b + c*d);
    dcm22 = aSq - bSq - cSq + dSq;

    % dcm_to_euler
    theta = asin(-dcm20);
    if abs(theta - d_pi2) < 1.0e-3
        phi = single(0.0);
        psi = atan2(dcm12, dcm02);
    elseif abs(theta + d_pi2) < 1.0e-3
        phi = single(0.0);
        psi = atan2(-dcm12, -dcm02);
    else
        phi = atan2(dcm21, dcm22);
        psi = atan2(dcm10, dcm00);
    end

end
